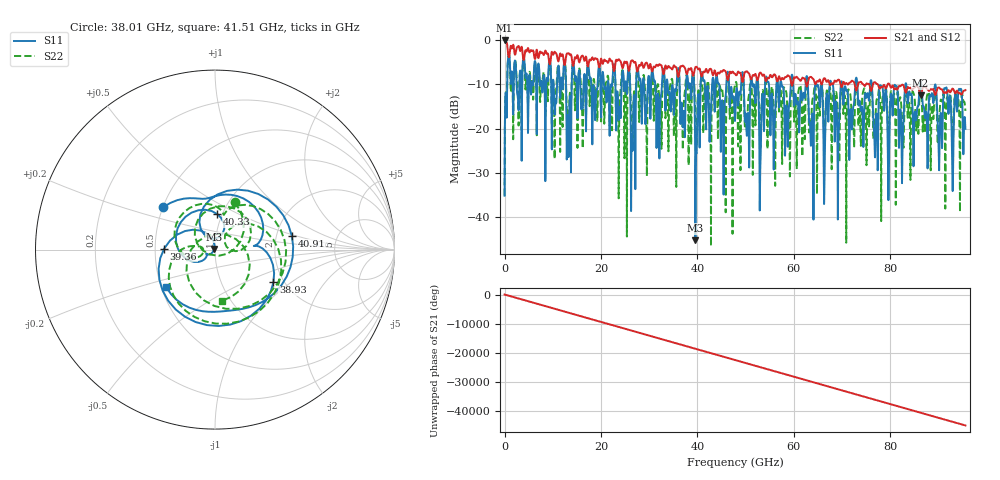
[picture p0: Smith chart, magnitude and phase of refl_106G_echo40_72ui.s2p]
! Created with skrf 1.10.0 (http://scikit-rf.org).
# GHz S RI R 50.0
!freq ReS11 ImS11 ReS21 ImS21 ReS12 ImS12 ReS22 ImS22
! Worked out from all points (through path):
!   3826 points, 10 MHz to 95.62 GHz, reference 50 ohm
!   highest |S21| = -0.06 dB at 10 MHz (marker M1); lowest = -12.5 dB at 86.33 GHz (marker M2)
!   group delay of S21, straight-line fit = 1.3 ns
!   lowest |S11| = -45.2 dB at 39.61 GHz (marker M3), VSWR 1.01, Z = 49.6 + j0.324 ohm
!   |S11| at or under -10 dB: 76.2 GHz to 83.18 GHz (6.976 GHz wide, 8.75 % of centre); 86.48 GHz to 89.34 GHz (2.859 GHz wide, 3.25 % of centre); 89.4 GHz to end of sweep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
!   |S22| runs from -46.5 to -3.2 dB; largest |S21 - S12| = 5.6e-16
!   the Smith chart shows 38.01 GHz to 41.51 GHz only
!   S11 on the Smith chart (normalised r, x): 38.01 GHz: 0.50, +0.27; 38.93 GHz: 1.76, -0.75; 39.36 GHz: 0.56, +0.01; 40.33 GHz: 0.95, +0.39; 40.91 GHz: 2.43, +0.47; 41.51 GHz: 0.53, -0.25
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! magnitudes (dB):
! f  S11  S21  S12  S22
! 10 MHz  -35.1  -0.1  -0.1  -35.1
! 1.06 GHz  -4.3  -2.9  -2.9  -4.5
! 15.96 GHz  -15.5  -3.6  -3.6  -12.4
! 31.88 GHz  -12.4  -5.8  -5.8  -10.2
! 38.01 GHz  -8.6  -7.1  -7.1  -10.9
! 38.93 GHz  -8.6  -7.4  -7.4  -9.6
! 39.36 GHz  -11.0  -7.1  -7.1  -9.8
! 39.61 GHz  -45.2  -6.1  -6.1  -18.4
! 40.33 GHz  -14.1  -6.5  -6.5  -12.1
! 40.91 GHz  -7.2  -8.2  -8.2  -8.2
! 41.51 GHz  -9.3  -7.2  -7.2  -10.9
! 47.83 GHz  -18.1  -7.6  -7.6  -10.1
! 62.53 GHz  -9.1  -9.8  -9.8  -10.7
! 63.75 GHz  -17.6  -8.5  -8.5  -15.2
! 67.83 GHz  -9.8  -9.8  -9.8  -23.7
! 68.9 GHz  -14.8  -9.3  -9.3  -12.1
! 75.83 GHz  -10.6  -10.7  -10.7  -12.4
! 77.08 GHz  -17.6  -9.7  -9.7  -14.6
! 78.13 GHz  -10.6  -10.5  -10.5  -32.0
! 79.7 GHz  -33.2  -9.8  -9.8  -24.2
! 86.33 GHz  -9.2  -12.5  -12.5  -10.1
! 95.62 GHz  -20.0  -11.3  -11.3  -16.0
